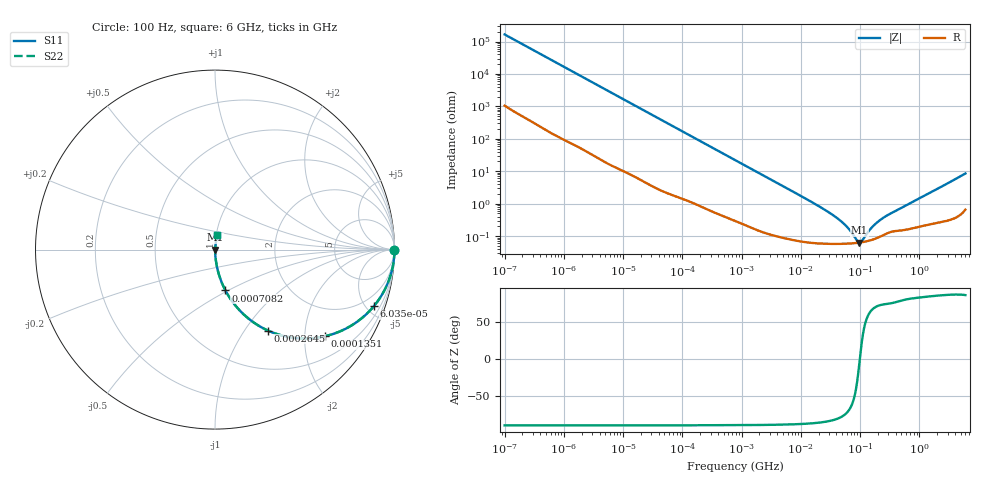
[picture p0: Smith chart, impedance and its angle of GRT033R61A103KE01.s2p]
!Murata Part Number: GRT033R61A103KE01
!These Parameters are Measured in Series Mode Connection
!Data Generated on Jun 19, 2026
!  o--ll--o
!Port1  Port2
!  o------o
!Operation Temp=25[degC], DC Bias Voltage=0[V]
!Freq. Start=100[Hz] Stop=6[GHz] 401[Steps]
# Hz S RI R 50
!Freq.(Hz) S11(Real) S11(Imag) S21(Real) S21(Imag) S12(Real) S12(Imag) S22(Real) S22(Imag)
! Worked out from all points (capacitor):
!   401 points, 100 Hz to 6 GHz, reference 50 ohm
!   read as one part in series: C = 9.61 nF near 109 Hz
!   lowest |Z| = 63.3 mohm at 97.54 MHz (marker M1)
!   series resonance near 99.2 MHz, so ESL is about 270 pH
!   S11 on the Smith chart (normalised r, x): 100 Hz: open; 60.35 kHz: 1.04, -5.60; 135.1 kHz: 1.02, -2.51; 264.5 kHz: 1.01, -1.29; 708.2 kHz: 1.01, -0.48; 6 GHz: 1.01, +0.17
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100  1 -0.000605  4.2e-06 0.000605  4.2e-06 0.000605  1 -0.000605
2008  0.9998 -0.012  0.000215 0.012  0.000215 0.012  0.9998 -0.012
12041  0.9945 -0.0712  0.00554 0.0712  0.00554 0.0712  0.9945 -0.0712
40335  0.9448 -0.2252  0.0552 0.2252  0.0552 0.2252  0.9448 -0.2252
60352  0.8853 -0.3151  0.1147 0.3151  0.1147 0.3151  0.8853 -0.3151
90302  0.7769 -0.4123  0.2231 0.4123  0.2231 0.4123  0.7769 -0.4123
135116  0.6113 -0.4829  0.3887 0.4829  0.3887 0.4829  0.6113 -0.4829
264476  0.2955 -0.4512  0.7045 0.4512  0.7045 0.4512  0.2955 -0.4512
413847  0.1486 -0.3501  0.8514 0.3501  0.8514 0.3501  0.1486 -0.3501
708247  0.0581 -0.2275  0.9419 0.2275  0.9419 0.2275  0.0581 -0.2275
774597  0.0494 -0.2101  0.9506 0.2101  0.9506 0.2101  0.0494 -0.2101
2594782  0.00563 -0.0663  0.9944 0.0663  0.9944 0.0663  0.00563 -0.0663
1.555665e7  0.000735 -0.011  0.9993 0.011  0.9993 0.011  0.000735 -0.011
4.764863e7  0.000584 -0.00283  0.9994 0.00283  0.9994 0.00283  0.000584 -0.00283
6.518806e7  0.00059 -0.00152  0.9994 0.00152  0.9994 0.00152  0.00059 -0.00152
8.918374e7  0.000617 -0.000375  0.9994 0.000375  0.9994 0.000375  0.000617 -0.000375
9.753859e7  0.00063 -5.86e-05  0.9994 5.86e-05  0.9994 5.86e-05  0.00063 -5.86e-05
1.066761e8  0.000645 0.000257  0.9994 -0.000257  0.9994 -0.000257  0.000645 0.000257
1.459435e8  0.000732 0.00138  0.9993 -0.00138  0.9993 -0.00138  0.000732 0.00138
1.825626e8  0.00084 0.00224  0.9992 -0.00224  0.9992 -0.00224  0.00084 0.00224
3.124326e8  0.00131 0.00455  0.9987 -0.00455  0.9987 -0.00455  0.00131 0.00455
6e9  0.0135 0.0834  0.9865 -0.0834  0.9865 -0.0834  0.0135 0.0834
